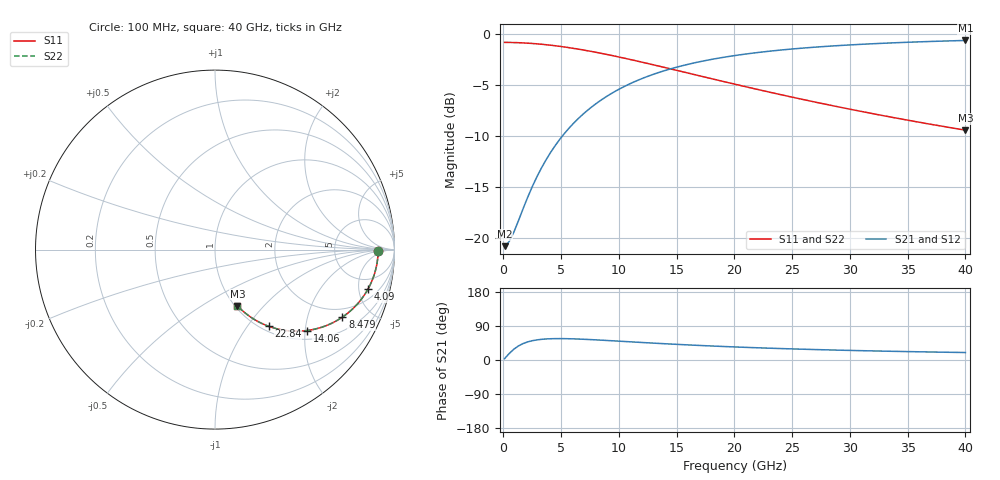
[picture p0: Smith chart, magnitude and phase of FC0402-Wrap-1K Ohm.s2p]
!Vishay Thin-Film
!FC Family
!Case Size 0402
!Assembly Style Full Wrap SMT
!10/21/2015
!thinfilm@vishay.com
# GHz S MA R 50
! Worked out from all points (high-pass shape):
!   101 points, 100 MHz to 40 GHz, reference 50 ohm
!   highest |S21| = -0.64 dB at 40 GHz (marker M1); lowest = -20.8 dB at 100 MHz (marker M2)
!   |S21| within 3 dB of the highest: 13.84 GHz to end of sweep
!   lowest |S11| = -9.4 dB at 40 GHz (marker M3), VSWR 2.02, Z = 51.3 - j36.3 ohm
!   |S11| at or under -10 dB: nowhere
!   |S22| runs from -9.4 to -0.8 dB; largest |S21 - S12| = 0
!   S11 on the Smith chart (normalised r, x): 100 MHz: 21, -1; 4.09 GHz: 3.24, -6.31; 8.479 GHz: 1.57, -3.33; 14.06 GHz: 1.21, -2.05; 22.84 GHz: 1.08, -1.27; 40 GHz: 1.03, -0.73
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0.1  0.9091 -0.4  0.09112 3.6  0.09112 3.6  0.9091 -0.4
0.499  0.9086 -1.8  0.09607 17.2  0.09607 17.2  0.9086 -1.8
0.898  0.9077 -3.2  0.1067 28.5  0.1067 28.5  0.9077 -3.2
2.095  0.9014 -7.5  0.1581 47.8  0.1581 47.8  0.9014 -7.5
2.494  0.8982 -8.9  0.1783 50.9  0.1783 50.9  0.8982 -8.9
3.292  0.8904 -11.6  0.2204 54.5  0.2204 54.5  0.8904 -11.6
4.09  0.8808 -14.3  0.2629 56.1  0.2629 56.1  0.8808 -14.3
5.287  0.8632 -18.3  0.3255 56.3  0.3255 56.3  0.8632 -18.3
6.085  0.8497 -20.8  0.3656 55.7  0.3656 55.7  0.8497 -20.8
6.883  0.8351 -23.3  0.404 54.8  0.404 54.8  0.8351 -23.3
8.479  0.8033 -27.9  0.4752 52.3  0.4752 52.3  0.8033 -27.9
9.676  0.7779 -31.2  0.5234 50.3  0.5234 50.3  0.7779 -31.2
10.873  0.7519 -34.2  0.5672 48.2  0.5672 48.2  0.7519 -34.2
13.666  0.6913 -40.5  0.6533 43.4  0.6533 43.4  0.6913 -40.5
14.065  0.6828 -41.3  0.6639 42.8  0.6639 42.8  0.6828 -41.3
16.858  0.6258 -46.5  0.7282 38.6  0.7282 38.6  0.6258 -46.5
20.05  0.567 -51.4  0.7839 34.4  0.7839 34.4  0.567 -51.4
22.843  0.5215 -55.0  0.8209 31.4  0.8209 31.4  0.5215 -55.0
26.833  0.4656 -59.2  0.8604 27.7  0.8604 27.7  0.4656 -59.2
30.025  0.4275 -62.0  0.8838 25.3  0.8838 25.3  0.4275 -62.0
33.616  0.3907 -64.6  0.904 23.0  0.904 23.0  0.3907 -64.6
40  0.3376 -68.2  0.9293 19.7  0.9293 19.7  0.3376 -68.2
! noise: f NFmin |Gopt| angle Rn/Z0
0.1  -7.232e-15  1  -1.207e-06  19.91
4.489  0  1  0  1.899
8.878  -4.822e-16  1  -6.298e-15  0.5221
13.27  0  1  -8.135e-15  0.2369
17.66  -4.822e-16  1  -1.606e-14  0.1342
22.05  0  1  -1.207e-06  0.08614
26.43  0  1  -8.538e-07  0.05984
30.82  0  1  -1.207e-06  0.04391
35.21  4.342e-09  1  -1.783e-14  0.03355
40  0  1  -1.708e-06  0.0259
